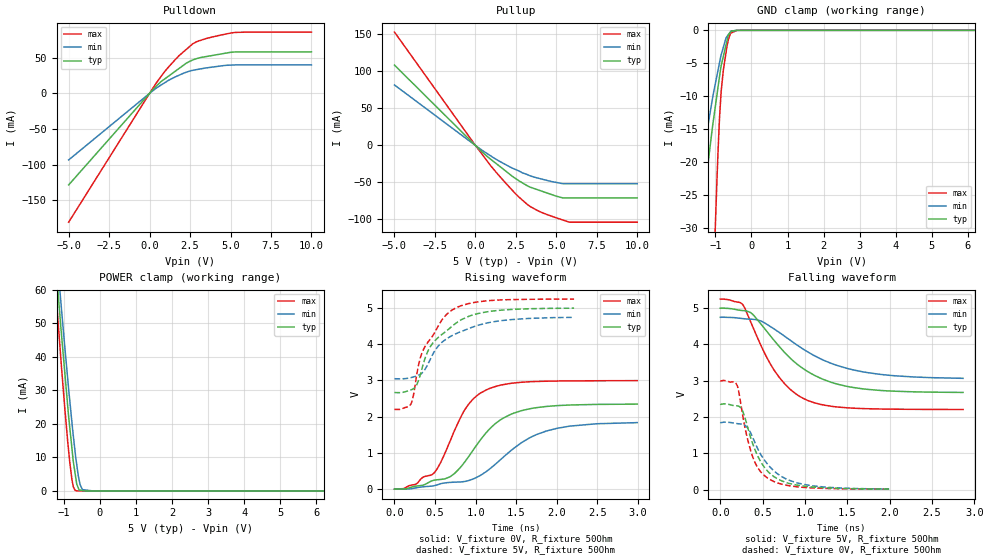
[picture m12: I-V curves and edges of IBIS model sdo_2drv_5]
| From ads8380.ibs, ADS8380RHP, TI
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|   sdo_2drv_5 Model
[Model]   sdo_2drv_5
Model_type   3-state
Polarity   Non-Inverting
Vmeas = 2.5
Vref = 2.5
Cref = 10pF
Rref = 50
|   typ   min   max
|   (nom PVT)   (fast PVT)   (slow PVT)
|C_comp from frequency sweep method (F=40MHz)
C_comp   5.189e-12   5.145e-12   5.197e-12
|ON state : BUFFER OUTPUT TURNED HIGH
|C_comp   4.653e-12   4.580e-12   4.708e-12
|OFF state: BUFFER IN HIGH IMPEDANCE
|C_comp   5.189e-12   5.145e-12   5.197e-12
|C_comp from LC tank measurement(L=1nH)
|Resonant Frequency(Hz)   4.130e+09   4.140e+09   4.100e+09
|C_comp   1.487e-12   1.479e-12   1.508e-12
|ON state : BUFFER OUTPUT TURNED HIGH
|Resonant Frequency(Hz)   4.130e+09   4.140e+09   4.100e+09
|C_comp   1.487e-12   1.479e-12   1.508e-12
|OFF state: BUFFER IN HIGH IMPEDANCE
|Resonant Frequency(Hz)   4.090e+09   4.100e+09   4.070e+09
|C_comp   1.516e-12   1.508e-12   1.531e-12
| Where nom  PVT is Nominal Process, 5V, 35C
|   Fast PVT is Strong Process,  5.25V, -40C
|   Slow PVT is Weak Process,   4.75V, 95C
[Voltage Range]   5   4.75   5.25
|Ambient Temperature   25   85   -40
|Junction Temperature
[Temperature Range]   35   95   -40
[Pullup Reference]   5   4.75   5.25
[Pulldown Reference]   0   0   0
[Power Clamp Reference]   5   4.75   5.25
[GND Clamp Reference]   0   0   0
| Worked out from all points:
|   slope of the pulldown table from 0 to 0.75 V, typ, clamps not added: 43.8 ohm
|   slope of the pullup table from 0 to 0.75 V, typ, clamps not added: 49 ohm
|   GND clamp passes 1 mA (typ) near -0.65 V on its own axis
|   POWER clamp passes 1 mA (typ) near -0.60 V on its own axis
|   falling waveform, V_fixture 5V, R_fixture 50Ohm: 20-80 % time 629ps typ, 761ps min, 447ps max; typ from 5 V to 2.68 V
|   rising waveform, V_fixture 0V, R_fixture 50Ohm: 20-80 % time 528ps typ, 664ps min, 398ps max; typ from 0 V to 2.35 V
|   rising waveform, V_fixture 5V, R_fixture 50Ohm: 20-80 % time 412ps typ, 485ps min, 325ps max; typ from 2.67 V to 4.99 V
|   falling waveform, V_fixture 0V, R_fixture 50Ohm: 20-80 % time 267ps typ, 335ps min, 201ps max; typ from 2.36 V to 0.011 V
[Pulldown]
|   Voltage   I(typ)   I(min)   I(max)
-5V       -128.3mA   -93.29mA   -180.5mA
420mV     10.19mA    7.351mA    14.75mA
924mV     20.01mA    14.71mA    30.2mA
1.596V    31.13mA    23.1mA     47.48mA
2.27V     42.28mA    29.65mA    61.58mA
2.672V    46.77mA    32.27mA    69.45mA
2.94V     48.89mA    33.38mA    72.7mA
3.433V    51.26mA    35.4mA     76.37mA
5.282V    57.95mA    39.81mA    85.33mA
10V       58.09mA    39.82mA    85.79mA
[GND Clamp]
|   Voltage   I(typ)   I(min)   I(max)
-5V       -615.5mA   -386.5mA   -1.626A
-1.64V    -41.74mA   -31.12mA   -149mA
-1.554V   -37.39mA   -27.67mA   -129.6mA
-1.31V    -25.06mA   -17.89mA   -83.47mA
-1.04V    -13.06mA   -9.152mA   -35.78mA
-955.5mV  -9.768mA   -6.844mA   -22.57mA
-892.5mV  -7.298mA   -5.113mA   -14.17mA
-840mV    -5.374mA   -3.735mA   -9.308mA
-777mV    -3.894mA   -2.533mA   -5.953mA
-677.3mV  -1.552mA   -932.8uA   -2.381mA
-565.3mV  -175.4uA   -114uA     -404uA
10V       0A         0A         0A
[Pullup]
|   Voltage   I(typ)   I(min)   I(max)
-5V       108.5mA    81.66mA    153.1mA
115.6fV   -57.8pA    -66.35pA   -45.68pA
924mV     -18.29mA   -13.84mA   -26.9mA
1.596V    -29.88mA   -22.71mA   -44.07mA
2.478V    -44.69mA   -32.52mA   -65.29mA
3.26V     -55.05mA   -39.92mA   -80.6mA
3.838V    -59.81mA   -43.99mA   -88.03mA
4.96V     -68.3mA    -49.85mA   -97.62mA
5.405V    -70.93mA   -51.7mA    -100.8mA
5.806V    -70.93mA   -51.7mA    -103.7mA
10V       -70.93mA   -51.7mA    -103.7mA
[POWER Clamp]
|   Voltage   I(typ)   I(min)   I(max)
-5V       1.111A     889.6mA    1.639A
-1.306V   79.05mA    85.45mA    71.92mA
-1.088V   49.82mA    57.38mA    40.53mA
-971.2mV  35.38mA    43.02mA    24.75mA
-829.5mV  18.56mA    26.58mA    8.235mA
-771.8mV  12.57mA    20.28mA    3.302mA
-687.7mV  5.414mA    11.93mA    186.9uA
-640mV    2.027mA    7.843mA    19.67uA
-546.3mV  251.2uA    1.859mA    2.402uA
-484.5mV  133.4uA    394.9uA    2.131uA
-190mV    0A         44.23nA    835.9nA
10V       0A         0A         0A
[Ramp]
R_load = 50
|   typ   min   max
dV/dt_r   1.41154/5.28441e-10   1.10857/6.71209e-10   1.80021/3.98086e-10
dV/dt_f   1.39963/6.34362e-10   1.0207/7.76622e-10   1.83006/4.49075e-10
[Falling Waveform]
V_fixture = 5V
V_fixture_min = 4.75V
V_fixture_max = 5.25V
R_fixture = 50Ohm
|   Time   V(typ)   V(min)   V(max)
0s        5V         4.75V      5.25V
264ps     4.936V     4.714V     5.103V
382ps     4.834V     4.695V     4.497V
524ps     4.437V     4.595V     3.759V
634ps     4.118V     4.431V     3.3V
808ps     3.665V     4.147V     2.803V
996ps     3.308V     3.848V     2.495V
1.316ns   2.953V     3.474V     2.294V
1.68ns    2.778V     3.248V     2.233V
2.868ns   2.677V     3.066V     2.206V
[Rising Waveform]
V_fixture = 0V
V_fixture_min = 0V
V_fixture_max = 0V
R_fixture = 50Ohm
|   Time   V(typ)   V(min)   V(max)
0s        4.571nV    8.364nV    3.948nV
264ps     83.68mV    36.32mV    137.8mV
490ps     247.4mV    96.11mV    453.9mV
688ps     347.3mV    187.2mV    1.341V
876ps     781.4mV    217.1mV    2.224V
990ps     1.145V     300.8mV    2.53V
1.162ns   1.638V     538.4mV    2.769V
1.44ns    2.07V      1.074V     2.92V
1.87ns    2.281V     1.603V     2.977V
2.99ns    2.345V     1.835V     2.993V
[Rising Waveform]
V_fixture = 5V
V_fixture_min = 4.75V
V_fixture_max = 5.25V
R_fixture = 50Ohm
|   Time   V(typ)   V(min)   V(max)
0s        2.665V     3.046V     2.199V
202ps     2.737V     3.075V     2.345V
234ps     2.768V     3.095V     2.595V
276ps     2.888V     3.124V     3.176V
346ps     3.386V     3.218V     3.799V
470ps     4.022V     3.713V     4.227V
594ps     4.284V     4.068V     4.696V
710ps     4.496V     4.236V     4.941V
1.156ns   4.896V     4.59V      5.197V
2.212ns   4.99V      4.738V     5.242V
[Falling Waveform]
V_fixture = 0V
V_fixture_min = 0V
V_fixture_max = 0V
R_fixture = 50Ohm
|   Time   V(typ)   V(min)   V(max)
0s        2.356V     1.852V     3.001V
200ps     2.308V     1.817V     2.867V
264ps     2.162V     1.796V     2.054V
302ps     1.893V     1.751V     1.592V
370ps     1.35V      1.505V     989.6mV
454ps     868.3mV    1.069V     561.6mV
570ps     480.1mV    666.2mV    298.7mV
724ps     239.7mV    358.2mV    148.8mV
926ps     113.3mV    171.3mV    69.17mV
1.996ns   11.34mV    12.98mV    9.557mV
